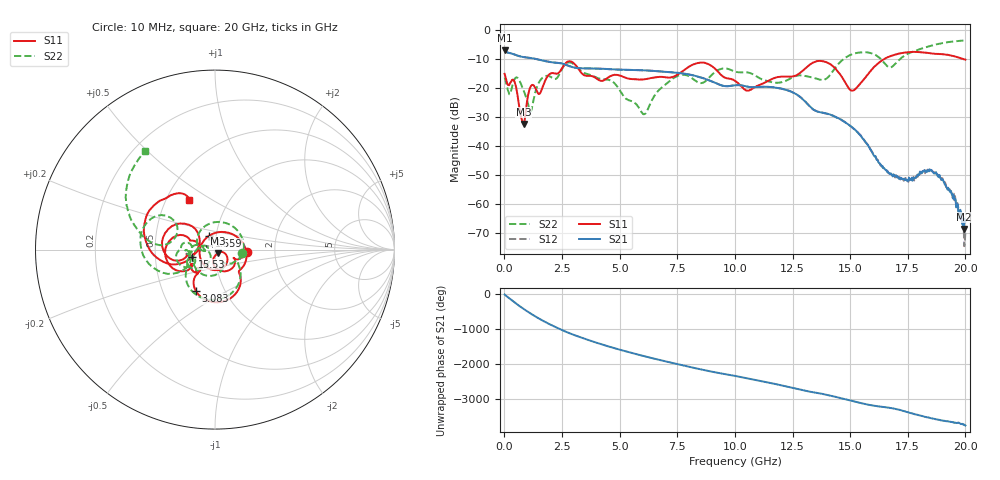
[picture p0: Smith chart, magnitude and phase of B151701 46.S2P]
!  2-Port S-parameters saved by WinCal
! VAR MeasName=S-Parameters (CALIBRATED_DATA) read from VNA (N5244A)
! VAR MeasDate=2015-12-24 19:14:53
! VAR NAME=B151701 46
! VAR FILENAME=B151701 46.S2P
! VAR DATE=2015-12-24 19:14:53
! VAR PHYS_PORTS=1,3
# Hz S DB R 50
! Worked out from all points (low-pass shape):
!   801 points, 10 MHz to 20 GHz, reference 50 ohm
!   highest |S21| = -6.87 dB at 10 MHz (marker M1); lowest = -68.5 dB at 19.93 GHz (marker M2)
!   |S21| within 3 dB of the highest: start of sweep to 1.376 GHz
!   lowest |S11| = -32.3 dB at 834.6 MHz (marker M3), VSWR 1.05, Z = 51.6 - j1.92 ohm
!   |S11| at or under -10 dB: start of sweep to 16.45 GHz; 19.96627 GHz to end of sweep
!   |S22| runs from -28.9 to -3.5 dB; largest |S21 - S12| = 0.0012
!   S11 on the Smith chart (normalised r, x): 10 MHz: 1.43, -0.04; 1.559 GHz: 0.92, +0.14; 3.083 GHz: 0.73, -0.36; 15.53 GHz: 0.77, -0.06; 20 GHz: 0.65, +0.40
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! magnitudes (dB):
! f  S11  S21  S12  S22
! 10 MHz  -15.0  -6.9  -6.9  -16.3
! 434.8 MHz  -17.6  -8.3  -8.3  -16.9
! 834.6 MHz  -32.3  -9.2  -9.2  -20.8
! 1.134 GHz  -19.4  -9.5  -9.5  -28.0
! 1.559 GHz  -21.6  -10.2  -10.2  -17.2
! 3.083 GHz  -11.9  -12.9  -12.9  -12.1
! 3.358 GHz  -14.8  -13.1  -13.1  -14.2
! 6.032 GHz  -16.9  -13.8  -13.8  -28.9
! 6.682 GHz  -16.1  -14.1  -14.1  -20.8
! 7.656 GHz  -14.5  -14.7  -14.7  -15.4
! 8.606 GHz  -11.1  -16.4  -16.4  -18.1
! 10.01 GHz  -17.4  -18.9  -18.9  -14.2
! 10.6 GHz  -20.8  -19.5  -19.5  -14.6
! 13.35 GHz  -11.3  -27.0  -27.0  -16.2
! 14.15 GHz  -11.7  -29.1  -29.1  -15.1
! 15.05 GHz  -20.8  -33.2  -33.3  -8.3
! 15.53 GHz  -17.5  -37.1  -37.1  -7.5
! 16.68 GHz  -9.1  -49.1  -49.4  -12.7
! 18.75 GHz  -8.1  -49.5  -49.7  -4.8
! 19.58 GHz  -9.0  -58.3  -59.0  -3.7
! 19.93 GHz  -9.9  -68.5  -67.3  -3.5
! 20 GHz  -10.1  -66.1  -69.4  -3.5
